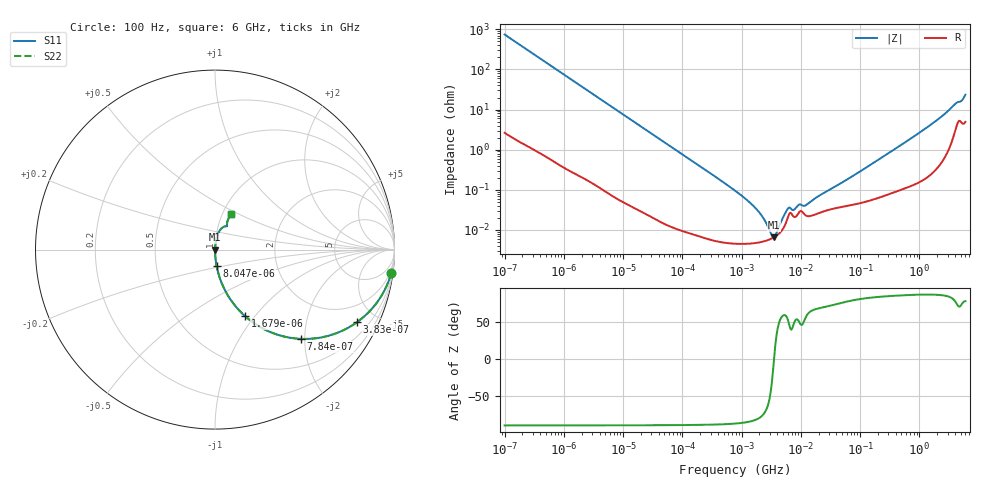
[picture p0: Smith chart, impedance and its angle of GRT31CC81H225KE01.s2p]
!Murata Part Number: GRT31CC81H225KE01
!These Parameters are Measured in Series Mode Connection
!Data Generated on Jun 19, 2026
!  o--ll--o
!Port1  Port2
!  o------o
!Operation Temp=25[degC], DC Bias Voltage=0[V]
!Freq. Start=100[Hz] Stop=6[GHz] 401[Steps]
# Hz S RI R 50
!Freq.(Hz) S11(Real) S11(Imag) S21(Real) S21(Imag) S12(Real) S12(Imag) S22(Real) S22(Imag)
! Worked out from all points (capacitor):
!   401 points, 100 Hz to 6 GHz, reference 50 ohm
!   read as one part in series: C = 2.13 uF near 109 Hz
!   lowest |Z| = 6.57 mohm at 3.55 MHz (marker M1)
!   series resonance near 3.531 MHz, so ESL is about 960 pH
!   S11 on the Smith chart (normalised r, x): 100 Hz: 1, -15; 383 Hz: 1.02, -3.91; 784 Hz: 1.01, -1.92; 1.679 kHz: 1.00, -0.90; 8.047 kHz: 1.00, -0.19; 6 GHz: 1.10, +0.46
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100  0.982 -0.1313  0.018 0.1313  0.018 0.1313  0.982 -0.1313
214  0.9236 -0.2637  0.0764 0.2637  0.0764 0.2637  0.9236 -0.2637
383  0.792 -0.4037  0.208 0.4037  0.208 0.4037  0.792 -0.4037
784  0.4788 -0.4973  0.5212 0.4973  0.5212 0.4973  0.4788 -0.4973
1679  0.1688 -0.372  0.8312 0.372  0.8312 0.372  0.1688 -0.372
2008  0.1248 -0.3278  0.8752 0.3278  0.8752 0.3278  0.1248 -0.3278
3594  0.0434 -0.2008  0.9566 0.2008  0.9566 0.2008  0.0434 -0.2008
8047  0.00935 -0.0932  0.9906 0.0932  0.9906 0.0932  0.00935 -0.0932
40335  0.000521 -0.0189  0.9995 0.0189  0.9995 0.0189  0.000521 -0.0189
774597  4.58e-05 -0.00095  1 0.00095  1 0.00095  4.58e-05 -0.00095
1734173  4.7e-05 -0.00034  1 0.00034  1 0.00034  4.7e-05 -0.00034
2967816  5.75e-05 -7.83e-05  0.9999 7.83e-05  0.9999 7.83e-05  5.75e-05 -7.83e-05
3549919  6.56e-05 2.5e-06  0.9999 -2.5e-06  0.9999 -2.5e-06  6.56e-05 2.5e-06
4246196  7.94e-05 8.66e-05  0.9999 -8.66e-05  0.9999 -8.66e-05  7.94e-05 8.66e-05
6075234  0.000209 0.000269  0.9998 -0.000269  0.9998 -0.000269  0.000209 0.000269
7599586  0.000212 0.000229  0.9998 -0.000229  0.9998 -0.000229  0.000212 0.000229
9506416  0.000283 0.000325  0.9997 -0.000325  0.9997 -0.000325  0.000283 0.000325
1.189169e7  0.000232 0.00033  0.9998 -0.00033  0.9998 -0.00033  0.000232 0.00033
1.555665e7  0.000227 0.000494  0.9998 -0.000494  0.9998 -0.000494  0.000227 0.000494
3.124326e8  0.000849 0.00839  0.9992 -0.00839  0.9992 -0.00839  0.000849 0.00839
1.95892e9  0.00613 0.0531  0.9939 -0.0531  0.9939 -0.0531  0.00613 0.0531
6e9  0.0905 0.1992  0.9095 -0.1992  0.9095 -0.1992  0.0905 0.1992
